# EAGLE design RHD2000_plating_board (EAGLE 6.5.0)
RHD2000 Evaluation Board

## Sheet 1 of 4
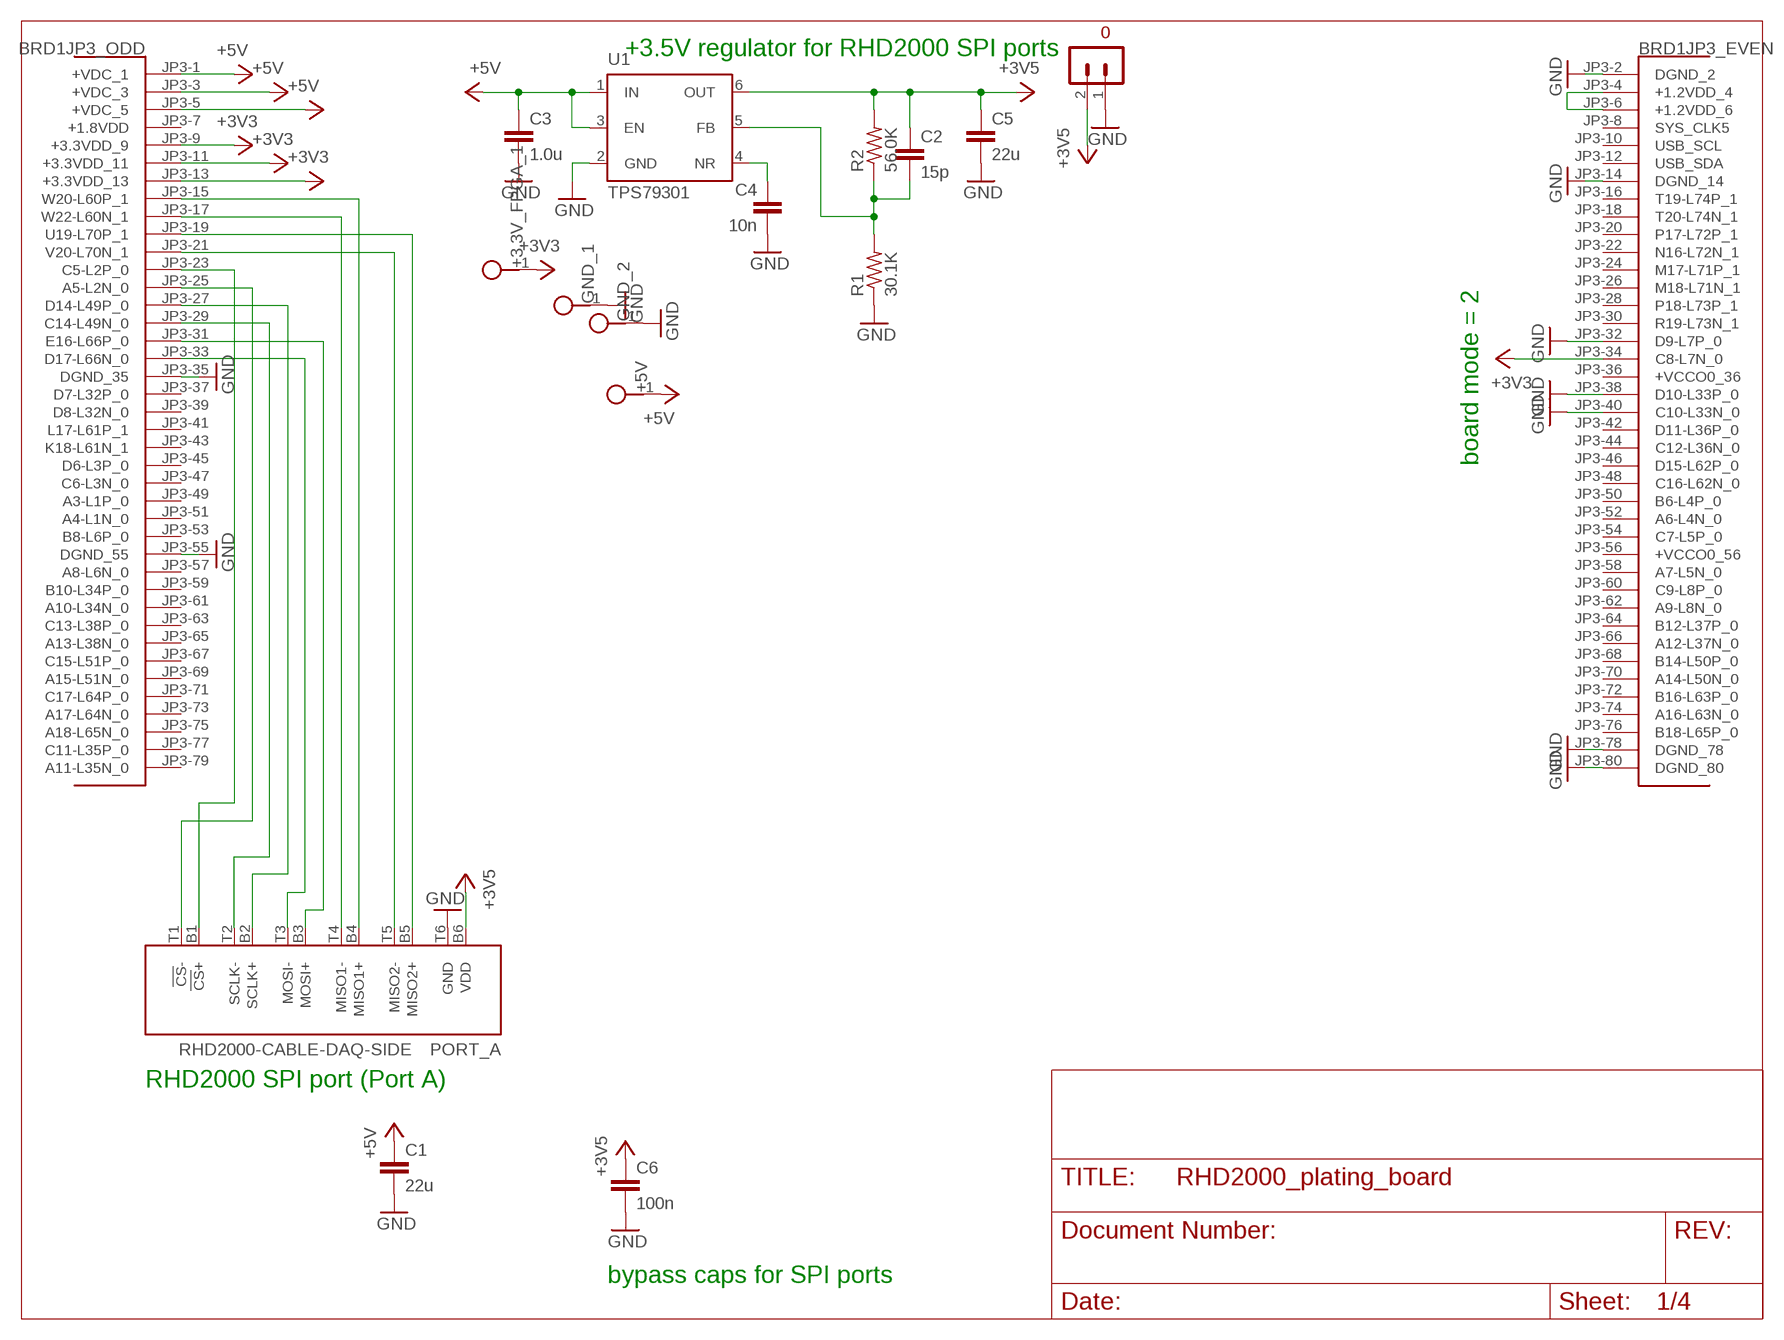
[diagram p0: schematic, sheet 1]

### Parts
+3.3V_FPGA_1  TESTPOINT  [TESTPOINT]
+5V  TESTPOINT  [TESTPOINT]
BRD1  OPALKELLY_XEM6010  [OPALKELLY_XEM6010]
C1  22u  C_1206  [1206]
C2  15p  C_0603  [0603]
C3  1.0u  C_0805  [0805]
C4  10n  C_0603  [0603]
C5  22u  C_1206  [1206]
C6  100n  C_0603  [0603]
GND_1  TESTPOINT  [TESTPOINT]
GND_2  TESTPOINT  [TESTPOINT]
PORT_A  RHD2000-CABLE-DAQ-SIDE  [OMNETICS_PZN-12-AA]
R1  30.1K  R_0603  [0603]
R2  56.0K  R_0603  [0603]
S2  TERMINAL_BLOCK_2-3.5MM-3.5V  [TERMINAL_BLOCK_3.5MM_2_3.5V]
U1  TPS79301  [SOT-23-6]

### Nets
+3V3 [power]: +3.3V_FPGA_1.1 BRD1.JP3-9(JP3_ODD:+3.3VDD_9) BRD1.JP3-11(JP3_ODD:+3.3VDD_11) BRD1.JP3-13(JP3_ODD:+3.3VDD_13) BRD1.JP3-34(JP3_EVEN:C8-L7N_0) ; also sheet 3
+3V5 [power]: C2.1 C5.1 C6.1 PORT_A.B6(VDD) R2.2 S2.2 U1.6(OUT)
+5V [power]: +5V.1 BRD1.JP3-1(JP3_ODD:+VDC_1) BRD1.JP3-3(JP3_ODD:+VDC_3) BRD1.JP3-5(JP3_ODD:+VDC_5) C1.1 C3.1 U1.1(IN) U1.3(EN) ; also sheet 4
GND [power]: BRD1.JP3-2(JP3_EVEN:DGND_2) BRD1.JP3-14(JP3_EVEN:DGND_14) BRD1.JP3-32(JP3_EVEN:D9-L7P_0) BRD1.JP3-35(JP3_ODD:DGND_35) BRD1.JP3-38(JP3_EVEN:D10-L33P_0) BRD1.JP3-40(JP3_EVEN:C10-L33N_0) BRD1.JP3-55(JP3_ODD:DGND_55) BRD1.JP3-78(JP3_EVEN:DGND_78) BRD1.JP3-80(JP3_EVEN:DGND_80) C1.2 C3.2 C4.2 C5.2 C6.2 GND_1.1 GND_2.1 PORT_A.T6(GND) R1.1 S2.1 U1.2(GND) ; also sheet 2,3,4
N$1: BRD1.JP3-15(JP3_ODD:W20-L60P_1) PORT_A.B4(MISO1+)
N$2: BRD1.JP3-17(JP3_ODD:W22-L60N_1) PORT_A.T4(MISO1-)
N$3: BRD1.JP3-19(JP3_ODD:U19-L70P_1) PORT_A.B5(MISO2+)
N$4: BRD1.JP3-21(JP3_ODD:V20-L70N_1) PORT_A.T5(MISO2-)
N$5: BRD1.JP3-23(JP3_ODD:C5-L2P_0) PORT_A.B1(!CS!+)
N$6: BRD1.JP3-25(JP3_ODD:A5-L2N_0) PORT_A.T1(!CS!-)
N$7: BRD1.JP3-27(JP3_ODD:D14-L49P_0) PORT_A.B2(SCLK+)
N$8: BRD1.JP3-29(JP3_ODD:C14-L49N_0) PORT_A.T2(SCLK-)
N$9: BRD1.JP3-31(JP3_ODD:E16-L66P_0) PORT_A.B3(MOSI+)
N$10: BRD1.JP3-33(JP3_ODD:D17-L66N_0) PORT_A.T3(MOSI-)
N$143: C4.1 U1.4(NR)
N$144: C2.2 R1.2 R2.1 U1.5(FB)
N$185 [power]: BRD1.JP3-4(JP3_EVEN:+1.2VDD_4) BRD1.JP3-6(JP3_EVEN:+1.2VDD_6)
Unconnected: BRD1.JP3-8(JP3_EVEN:SYS_CLK5) BRD1.JP3-10(JP3_EVEN:USB_SCL) BRD1.JP3-12(JP3_EVEN:USB_SDA) BRD1.JP3-16(JP3_EVEN:T19-L74P_1) BRD1.JP3-18(JP3_EVEN:T20-L74N_1) BRD1.JP3-20(JP3_EVEN:P17-L72P_1) BRD1.JP3-22(JP3_EVEN:N16-L72N_1) BRD1.JP3-24(JP3_EVEN:M17-L71P_1) BRD1.JP3-26(JP3_EVEN:M18-L71N_1) BRD1.JP3-28(JP3_EVEN:P18-L73P_1) BRD1.JP3-30(JP3_EVEN:R19-L73N_1) BRD1.JP3-37(JP3_ODD:D7-L32P_0) BRD1.JP3-39(JP3_ODD:D8-L32N_0) BRD1.JP3-41(JP3_ODD:L17-L61P_1) BRD1.JP3-42(JP3_EVEN:D11-L36P_0) BRD1.JP3-43(JP3_ODD:K18-L61N_1) BRD1.JP3-44(JP3_EVEN:C12-L36N_0) BRD1.JP3-45(JP3_ODD:D6-L3P_0) BRD1.JP3-46(JP3_EVEN:D15-L62P_0) BRD1.JP3-47(JP3_ODD:C6-L3N_0) BRD1.JP3-48(JP3_EVEN:C16-L62N_0) BRD1.JP3-49(JP3_ODD:A3-L1P_0) BRD1.JP3-50(JP3_EVEN:B6-L4P_0) BRD1.JP3-51(JP3_ODD:A4-L1N_0) BRD1.JP3-52(JP3_EVEN:A6-L4N_0) BRD1.JP3-53(JP3_ODD:B8-L6P_0) BRD1.JP3-54(JP3_EVEN:C7-L5P_0) BRD1.JP3-57(JP3_ODD:A8-L6N_0) BRD1.JP3-58(JP3_EVEN:A7-L5N_0) BRD1.JP3-59(JP3_ODD:B10-L34P_0) BRD1.JP3-60(JP3_EVEN:C9-L8P_0) BRD1.JP3-61(JP3_ODD:A10-L34N_0) BRD1.JP3-62(JP3_EVEN:A9-L8N_0) BRD1.JP3-63(JP3_ODD:C13-L38P_0) BRD1.JP3-64(JP3_EVEN:B12-L37P_0) BRD1.JP3-65(JP3_ODD:A13-L38N_0) BRD1.JP3-66(JP3_EVEN:A12-L37N_0) BRD1.JP3-67(JP3_ODD:C15-L51P_0) BRD1.JP3-68(JP3_EVEN:B14-L50P_0) BRD1.JP3-69(JP3_ODD:A15-L51N_0) BRD1.JP3-70(JP3_EVEN:A14-L50N_0) BRD1.JP3-71(JP3_ODD:C17-L64P_0) BRD1.JP3-72(JP3_EVEN:B16-L63P_0) BRD1.JP3-73(JP3_ODD:A17-L64N_0) BRD1.JP3-74(JP3_EVEN:A16-L63N_0) BRD1.JP3-75(JP3_ODD:A18-L65N_0) BRD1.JP3-76(JP3_EVEN:B18-L65P_0) BRD1.JP3-77(JP3_ODD:C11-L35P_0) BRD1.JP3-79(JP3_ODD:A11-L35N_0)

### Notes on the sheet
- +3.5V regulator for RHD2000 SPI ports
- board mode = 2
- RHD2000 SPI port (Port A)
- bypass caps for SPI ports

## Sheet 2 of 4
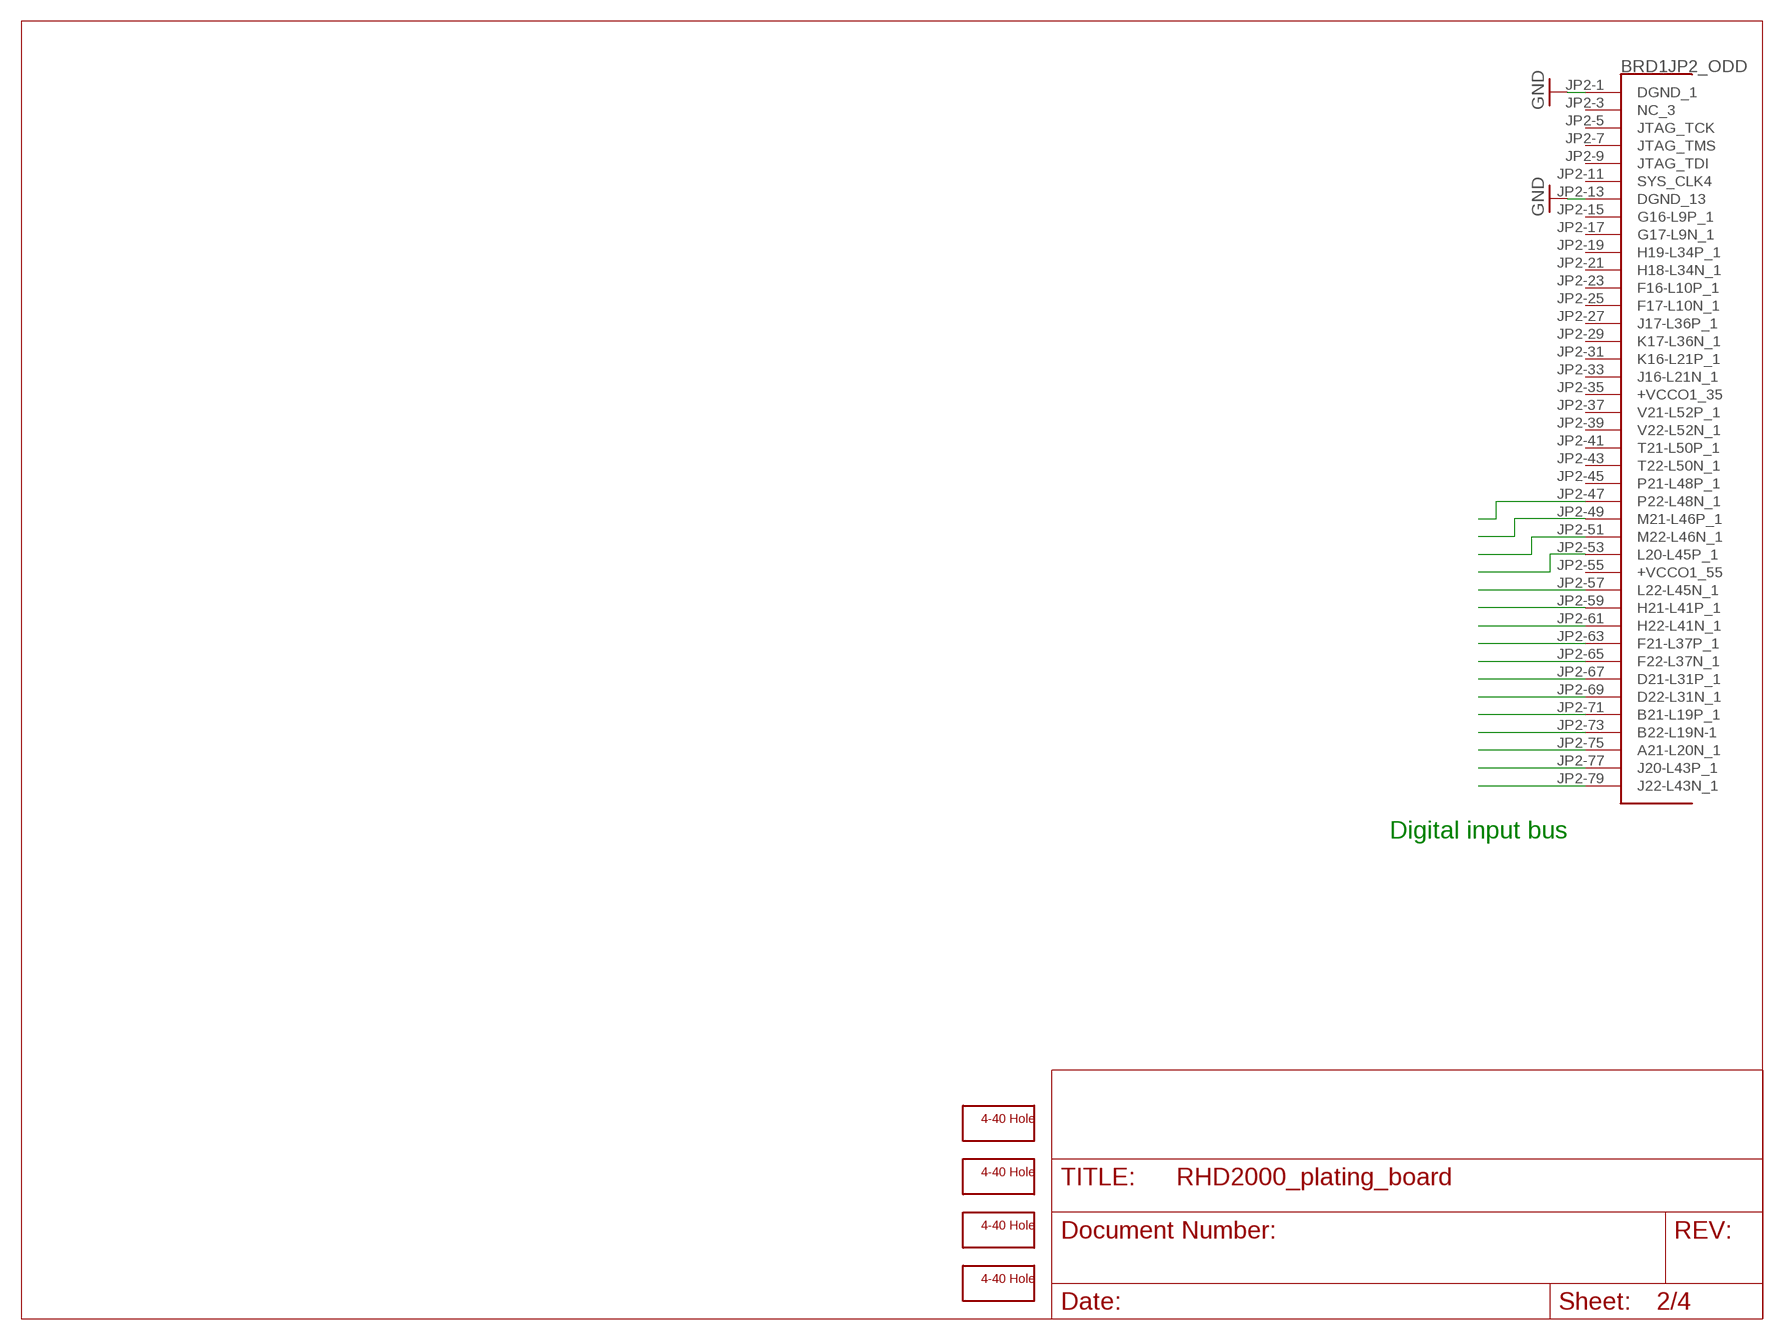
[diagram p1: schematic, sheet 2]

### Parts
H1  SCREW_HOLE_4-40  [SCREW_HOLE_4-40]
H2  SCREW_HOLE_4-40  [SCREW_HOLE_4-40]
H3  SCREW_HOLE_4-40  [SCREW_HOLE_4-40]
H4  SCREW_HOLE_4-40  [SCREW_HOLE_4-40]

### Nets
GND [power]: BRD1.JP2-1(JP2_ODD:DGND_1) BRD1.JP2-13(JP2_ODD:DGND_13) ; also sheet 1,3,4
N$68: BRD1.JP2-79(JP2_ODD:J22-L43N_1)
N$69: BRD1.JP2-77(JP2_ODD:J20-L43P_1)
N$70: BRD1.JP2-75(JP2_ODD:A21-L20N_1)
N$71: BRD1.JP2-73(JP2_ODD:B22-L19N-1)
N$72: BRD1.JP2-71(JP2_ODD:B21-L19P_1)
N$73: BRD1.JP2-69(JP2_ODD:D22-L31N_1)
N$74: BRD1.JP2-67(JP2_ODD:D21-L31P_1)
N$75: BRD1.JP2-65(JP2_ODD:F22-L37N_1)
N$76: BRD1.JP2-63(JP2_ODD:F21-L37P_1)
N$77: BRD1.JP2-61(JP2_ODD:H22-L41N_1)
N$78: BRD1.JP2-59(JP2_ODD:H21-L41P_1)
N$79: BRD1.JP2-57(JP2_ODD:L22-L45N_1)
N$80: BRD1.JP2-53(JP2_ODD:L20-L45P_1)
N$81: BRD1.JP2-51(JP2_ODD:M22-L46N_1)
N$82: BRD1.JP2-49(JP2_ODD:M21-L46P_1)
N$83: BRD1.JP2-47(JP2_ODD:P22-L48N_1)
Unconnected: BRD1.JP2-3(JP2_ODD:NC_3) BRD1.JP2-5(JP2_ODD:JTAG_TCK) BRD1.JP2-7(JP2_ODD:JTAG_TMS) BRD1.JP2-9(JP2_ODD:JTAG_TDI) BRD1.JP2-11(JP2_ODD:SYS_CLK4) BRD1.JP2-15(JP2_ODD:G16-L9P_1) BRD1.JP2-17(JP2_ODD:G17-L9N_1) BRD1.JP2-19(JP2_ODD:H19-L34P_1) BRD1.JP2-21(JP2_ODD:H18-L34N_1) BRD1.JP2-23(JP2_ODD:F16-L10P_1) BRD1.JP2-25(JP2_ODD:F17-L10N_1) BRD1.JP2-27(JP2_ODD:J17-L36P_1) BRD1.JP2-29(JP2_ODD:K17-L36N_1) BRD1.JP2-31(JP2_ODD:K16-L21P_1) BRD1.JP2-33(JP2_ODD:J16-L21N_1) BRD1.JP2-37(JP2_ODD:V21-L52P_1) BRD1.JP2-39(JP2_ODD:V22-L52N_1) BRD1.JP2-41(JP2_ODD:T21-L50P_1) BRD1.JP2-43(JP2_ODD:T22-L50N_1) BRD1.JP2-45(JP2_ODD:P21-L48P_1)

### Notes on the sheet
- Digital input bus

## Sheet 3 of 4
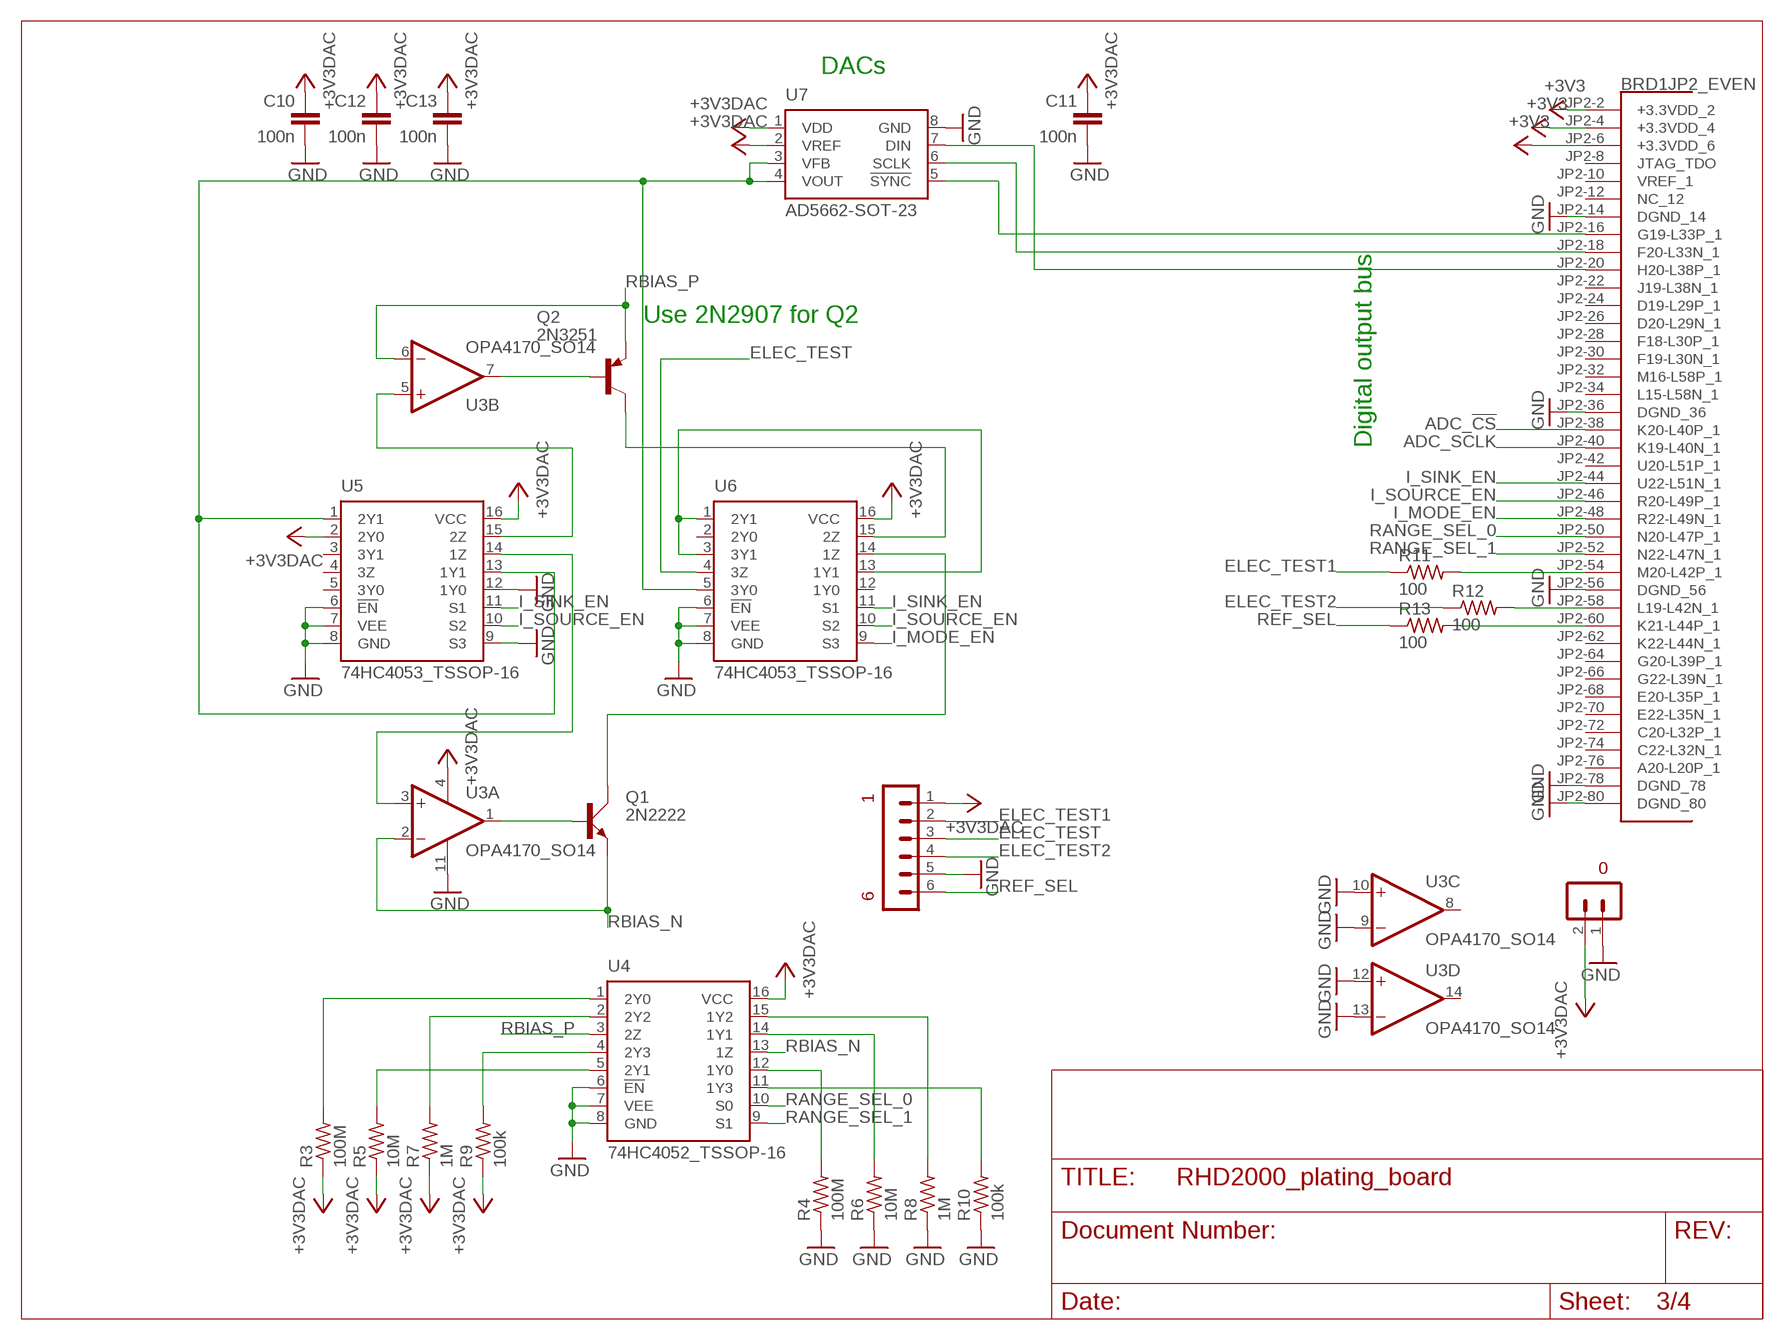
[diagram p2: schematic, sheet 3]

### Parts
C10  100n  C_0603  [0603]
C11  100n  C_0603  [0603]
C12  100n  C_0603  [0603]
C13  100n  C_0603  [0603]
Q1  2N2222  [TO18A]
Q2  2N3251  [TO18]
R3  100M  R_1206  [1206]
R4  100M  R_1206  [1206]
R5  10M  R_0603  [0603]
R6  10M  R_0603  [0603]
R7  1M  R_0603  [0603]
R8  1M  R_0603  [0603]
R9  100k  R_0603  [0603]
R10  100k  R_0603  [0603]
R11  100  R_0603  [0603]
R12  100  R_0603  [0603]
R13  100  R_0603  [0603]
S1  TERMINAL_BLOCK_2-3.5MM-3.3V  [TERMINAL_BLOCK_3.5MM_2_3.3V]
S3  WIRES-6  [WIRES-6]
U3  OPA4170_SO14  [SOIC-14]
U4  74HC4052_TSSOP-16  [TSSOP-16]
U5  74HC4053_TSSOP-16  [TSSOP-16]
U6  74HC4053_TSSOP-16  [TSSOP-16]
U7  AD5662-SOT-23  [SOT-23-RJ-8]

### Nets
+3V3 [power]: BRD1.JP2-2(JP2_EVEN:+3.3VDD_2) BRD1.JP2-4(JP2_EVEN:+3.3VDD_4) BRD1.JP2-6(JP2_EVEN:+3.3VDD_6) ; also sheet 1
+3V3DAC [power]: C10.1 C11.1 C12.1 C13.1 R3.1 R5.1 R7.1 R9.1 S1.2 S3.1 U3.4(P:V+) U4.16(VCC) U5.2(2Y0) U5.16(VCC) U6.16(VCC) U7.1(VDD) U7.2(VREF) ; also sheet 4
ADC_!CS!: BRD1.JP2-38(JP2_EVEN:K20-L40P_1)
ADC_SCLK: BRD1.JP2-40(JP2_EVEN:K19-L40N_1)
ELEC_TEST: S3.3 U6.4(3Z)
ELEC_TEST1: R11.1 S3.2
ELEC_TEST2: R12.1 S3.4
GND [power]: BRD1.JP2-14(JP2_EVEN:DGND_14) BRD1.JP2-36(JP2_EVEN:DGND_36) BRD1.JP2-56(JP2_EVEN:DGND_56) BRD1.JP2-78(JP2_EVEN:DGND_78) BRD1.JP2-80(JP2_EVEN:DGND_80) C10.2 C11.2 C12.2 C13.2 R4.1 R6.1 R8.1 R10.1 S1.1 S3.5 U3.9(C:-IN) U3.10(C:+IN) U3.11(P:V-) U3.12(D:+IN) U3.13(D:-IN) U4.6(!EN!) U4.7(VEE) U4.8(GND) U5.6(!EN!) U5.7(VEE) U5.8(GND) U5.9(S3) U5.12(1Y0) U6.6(!EN!) U6.7(VEE) U6.8(GND) U7.8(GND) ; also sheet 1,2,4
I_MODE_EN: BRD1.JP2-48(JP2_EVEN:R22-L49N_1) U6.9(S3)
I_SINK_EN: BRD1.JP2-44(JP2_EVEN:U22-L51N_1) U5.11(S1) U6.11(S1)
I_SOURCE_EN: BRD1.JP2-46(JP2_EVEN:R20-L49P_1) U5.10(S2) U6.10(S2)
N$11: Q1.B U3.1(A:OUT)
N$12: U5.1(2Y1) U5.13(1Y1) U6.5(3Y0) U7.3(VFB) U7.4(VOUT)
N$13: U3.3(A:+IN) U5.14(1Z)
N$14: Q1.C U6.14(1Z)
N$15: U3.5(B:+IN) U5.15(2Z)
N$16: Q2.2(B) U3.7(B:OUT)
N$17: Q2.3(C) U6.15(2Z)
N$18: BRD1.JP2-54(JP2_EVEN:M20-L42P_1) R11.2
N$19: BRD1.JP2-58(JP2_EVEN:L19-L42N_1) R12.2
N$20: R9.2 U4.4(2Y3)
N$21: R7.2 U4.2(2Y2)
N$22: R5.2 U4.5(2Y1)
N$23: R3.2 U4.1(2Y0)
N$24: R4.2 U4.12(1Y0)
N$25: R6.2 U4.14(1Y1)
N$26: R8.2 U4.15(1Y2)
N$27: R10.2 U4.11(1Y3)
N$28: U6.1(2Y1) U6.3(3Y1) U6.13(1Y1)
N$29: BRD1.JP2-60(JP2_EVEN:K21-L44P_1) R13.2
N$41: BRD1.JP2-16(JP2_EVEN:G19-L33P_1) U7.5(!SYNC!)
N$42: BRD1.JP2-18(JP2_EVEN:F20-L33N_1) U7.6(SCLK)
N$43: BRD1.JP2-20(JP2_EVEN:H20-L38P_1) U7.7(DIN)
RANGE_SEL_0: BRD1.JP2-50(JP2_EVEN:N20-L47P_1) U4.10(S0)
RANGE_SEL_1: BRD1.JP2-52(JP2_EVEN:N22-L47N_1) U4.9(S1)
RBIAS_N: Q1.E U3.2(A:-IN) U4.13(1Z)
RBIAS_P: Q2.1(E) U3.6(B:-IN) U4.3(2Z)
REF_SEL: R13.1 S3.6
Unconnected: BRD1.JP2-8(JP2_EVEN:JTAG_TDO) BRD1.JP2-10(JP2_EVEN:VREF_1) BRD1.JP2-12(JP2_EVEN:NC_12) BRD1.JP2-22(JP2_EVEN:J19-L38N_1) BRD1.JP2-24(JP2_EVEN:D19-L29P_1) BRD1.JP2-26(JP2_EVEN:D20-L29N_1) BRD1.JP2-28(JP2_EVEN:F18-L30P_1) BRD1.JP2-30(JP2_EVEN:F19-L30N_1) BRD1.JP2-32(JP2_EVEN:M16-L58P_1) BRD1.JP2-34(JP2_EVEN:L15-L58N_1) BRD1.JP2-42(JP2_EVEN:U20-L51P_1) BRD1.JP2-62(JP2_EVEN:K22-L44N_1) BRD1.JP2-64(JP2_EVEN:G20-L39P_1) BRD1.JP2-66(JP2_EVEN:G22-L39N_1) BRD1.JP2-68(JP2_EVEN:E20-L35P_1) BRD1.JP2-70(JP2_EVEN:E22-L35N_1) BRD1.JP2-72(JP2_EVEN:C20-L32P_1) BRD1.JP2-74(JP2_EVEN:C22-L32N_1) BRD1.JP2-76(JP2_EVEN:A20-L20P_1) U3.8(C:OUT) U3.14(D:OUT) U5.3(3Y1) U5.4(3Z) U5.5(3Y0) U6.2(2Y0) U6.12(1Y0)

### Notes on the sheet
- DACs
- Use 2N2907 for Q2
- Digital output bus

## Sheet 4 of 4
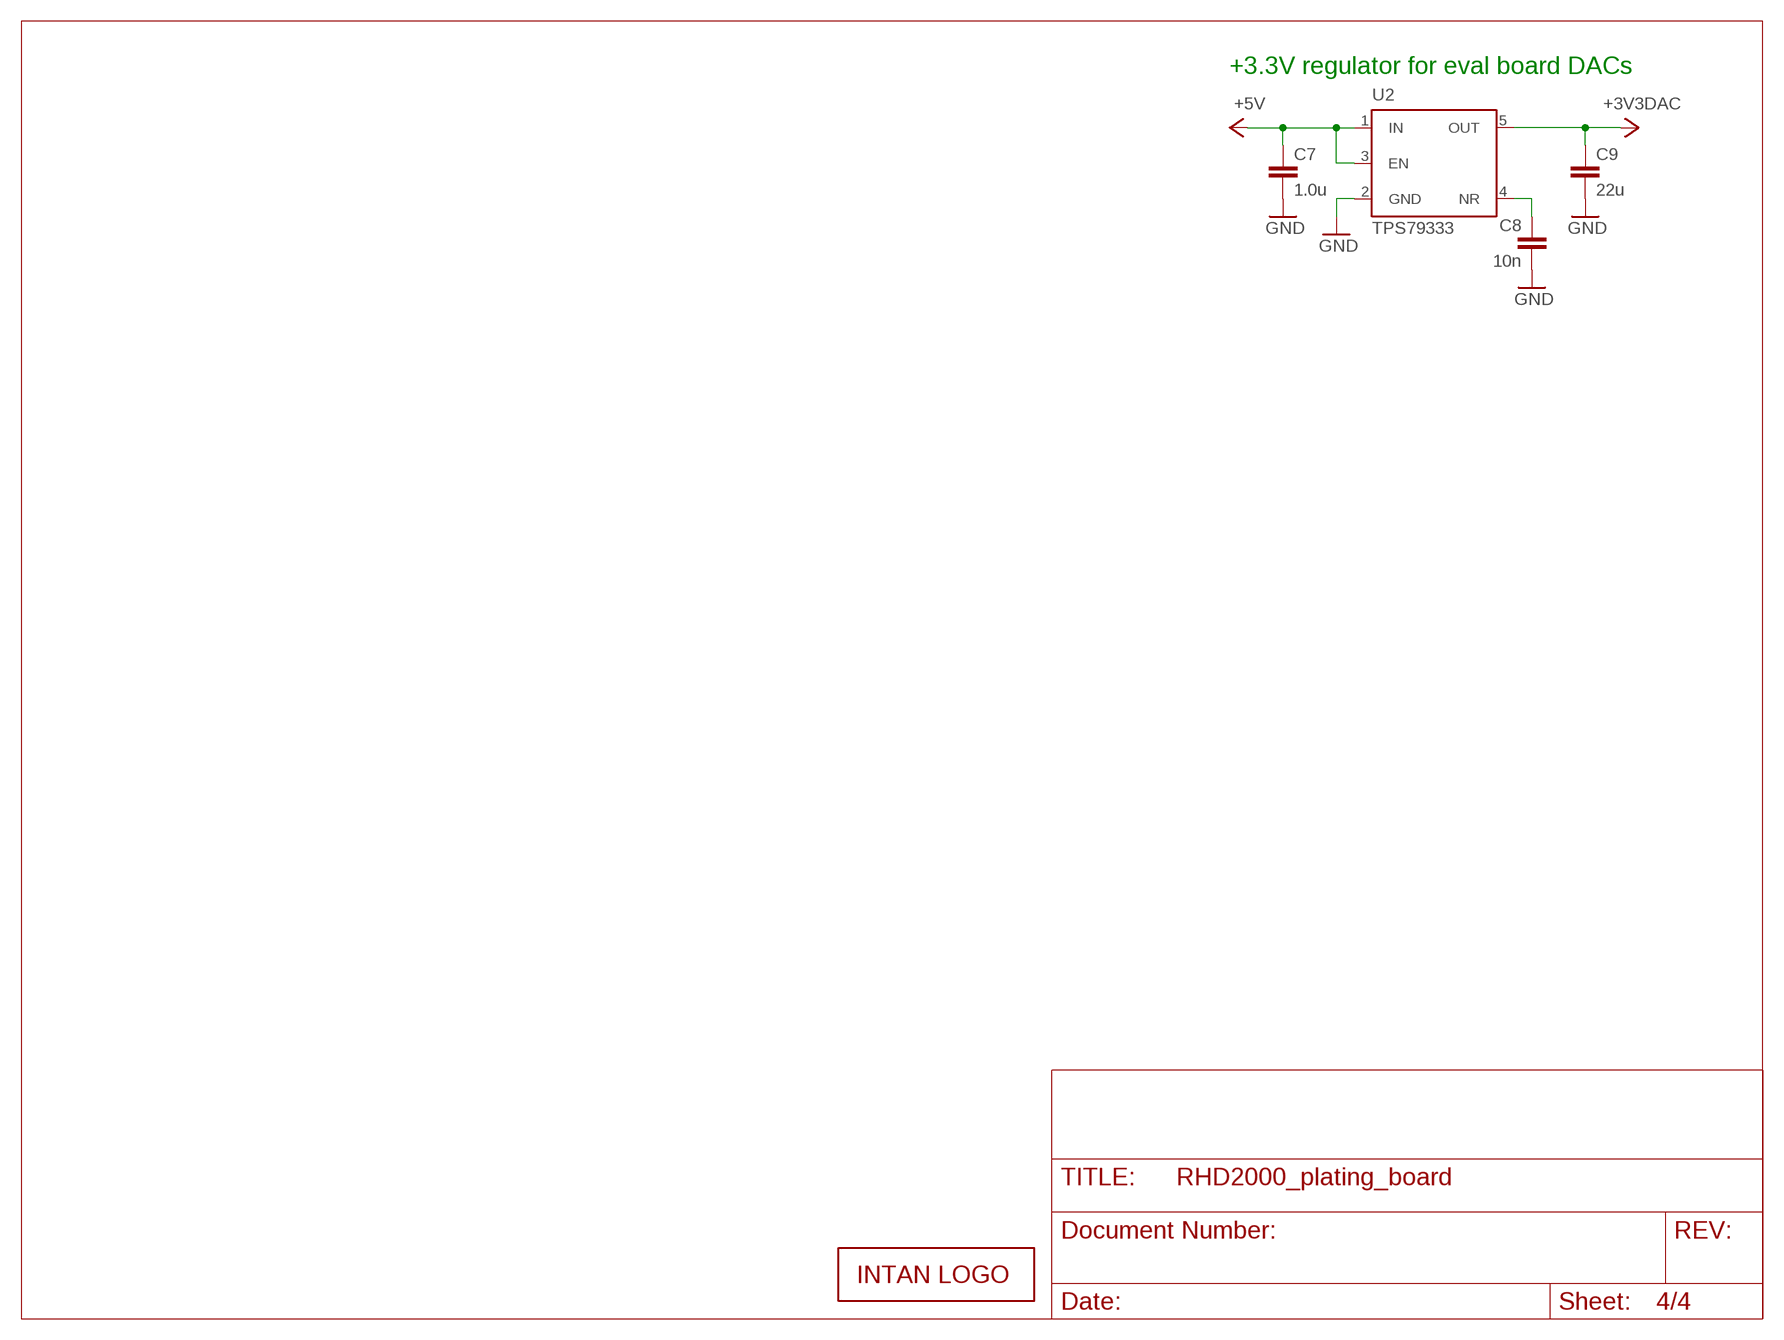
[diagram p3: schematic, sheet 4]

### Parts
C7  1.0u  C_0805  [0805]
C8  10n  C_0603  [0603]
C9  22u  C_1206  [1206]
LOGO1  INTAN_LOGO  [INTAN_LOGO]
U2  TPS79333  [SOT-23-5]

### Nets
+3V3DAC [power]: C9.1 U2.5(OUT) ; also sheet 3
+5V [power]: C7.1 U2.1(IN) U2.3(EN) ; also sheet 1
GND [power]: C7.2 C8.2 C9.2 U2.2(GND) ; also sheet 1,2,3
N$141: C8.1 U2.4(NR)

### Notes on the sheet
- +3.3V regulator for eval board DACs

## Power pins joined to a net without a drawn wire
+1.8VDD: BRD1.JP3-7(JP3_ODD:+1.8VDD)
+VCCO0_36: BRD1.JP3-36(JP3_EVEN:+VCCO0_36)
+VCCO0_56: BRD1.JP3-56(JP3_EVEN:+VCCO0_56)
+VCCO1_35: BRD1.JP2-35(JP2_ODD:+VCCO1_35)
+VCCO1_55: BRD1.JP2-55(JP2_ODD:+VCCO1_55)

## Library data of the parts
+3.3V_FPGA_1 +5V GND_1 GND_2 = RHD2000_eval_board:TESTPOINT: PCB Test Point
BRD1 = RHD2000_eval_board:OPALKELLY_XEM6010: Opal Kelly XEM6010 USB/FPGA module
C1-C13 = RHD2000_eval_board:C: Capacitor
H1-H4 = RHD2000_eval_board:SCREW_HOLE_4-40: Mounting hole
LOGO1 = RHD2000_eval_board:INTAN_LOGO
PORT_A = RHD2000_eval_board:RHD2000-CABLE-DAQ-SIDE: Omnetics PZN-12-AA RHD2000 socket - DAQ side
Q1 = transistor-small-signal:2N2222: NPN TRANSISTOR
Q2 = transistor-pnp:2N3251: PNP Transistror
R1-R13 = RHD2000_eval_board:R: Resistor
S1 S2 = RHD2000_eval_board:TERMINAL_BLOCK_2: 2-point terminal block
S3 = harrison:WIRES-6
U1 = RHD2000_eval_board:TPS79301: Texas Instruments TPS79301 adjustable regulator
U2 = RHD2000_eval_board:TPS79333: Texas Instruments TPS79333 3.3V LDO regulator
U3 = RHD2000_eval_board:OPA4170: TI OPA4170 quad op amp
U4 = harrison:74HC4052
U5 U6 = harrison:74HC4053
U7 = RHD2000_eval_board:AD5662: Analog Devices AD5662 16-bit DAC

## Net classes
1 power: width 0.381 mm

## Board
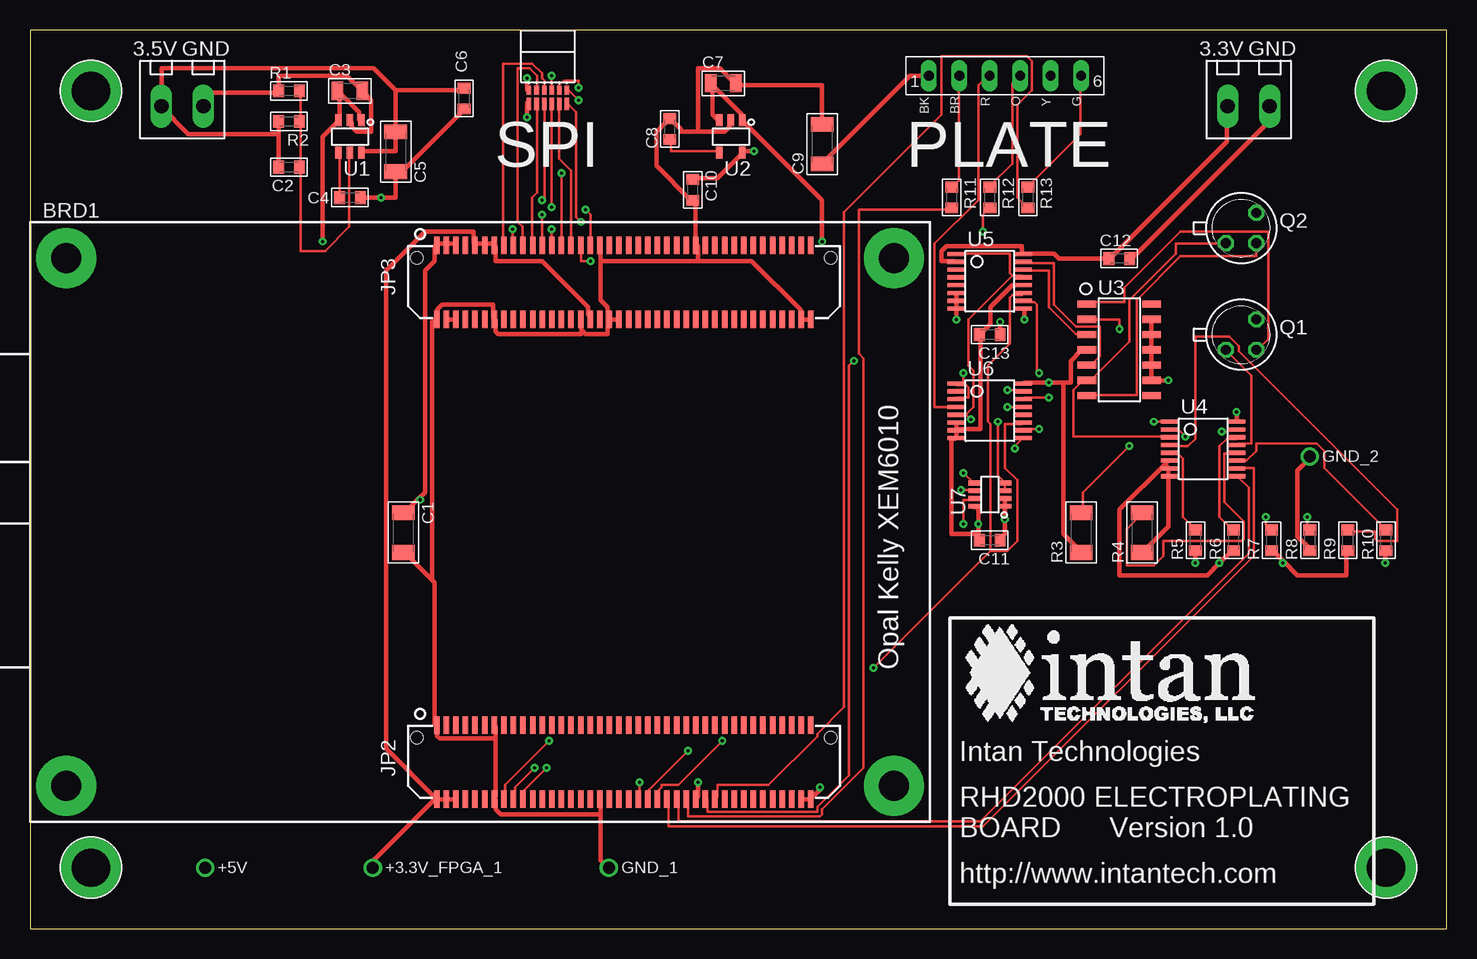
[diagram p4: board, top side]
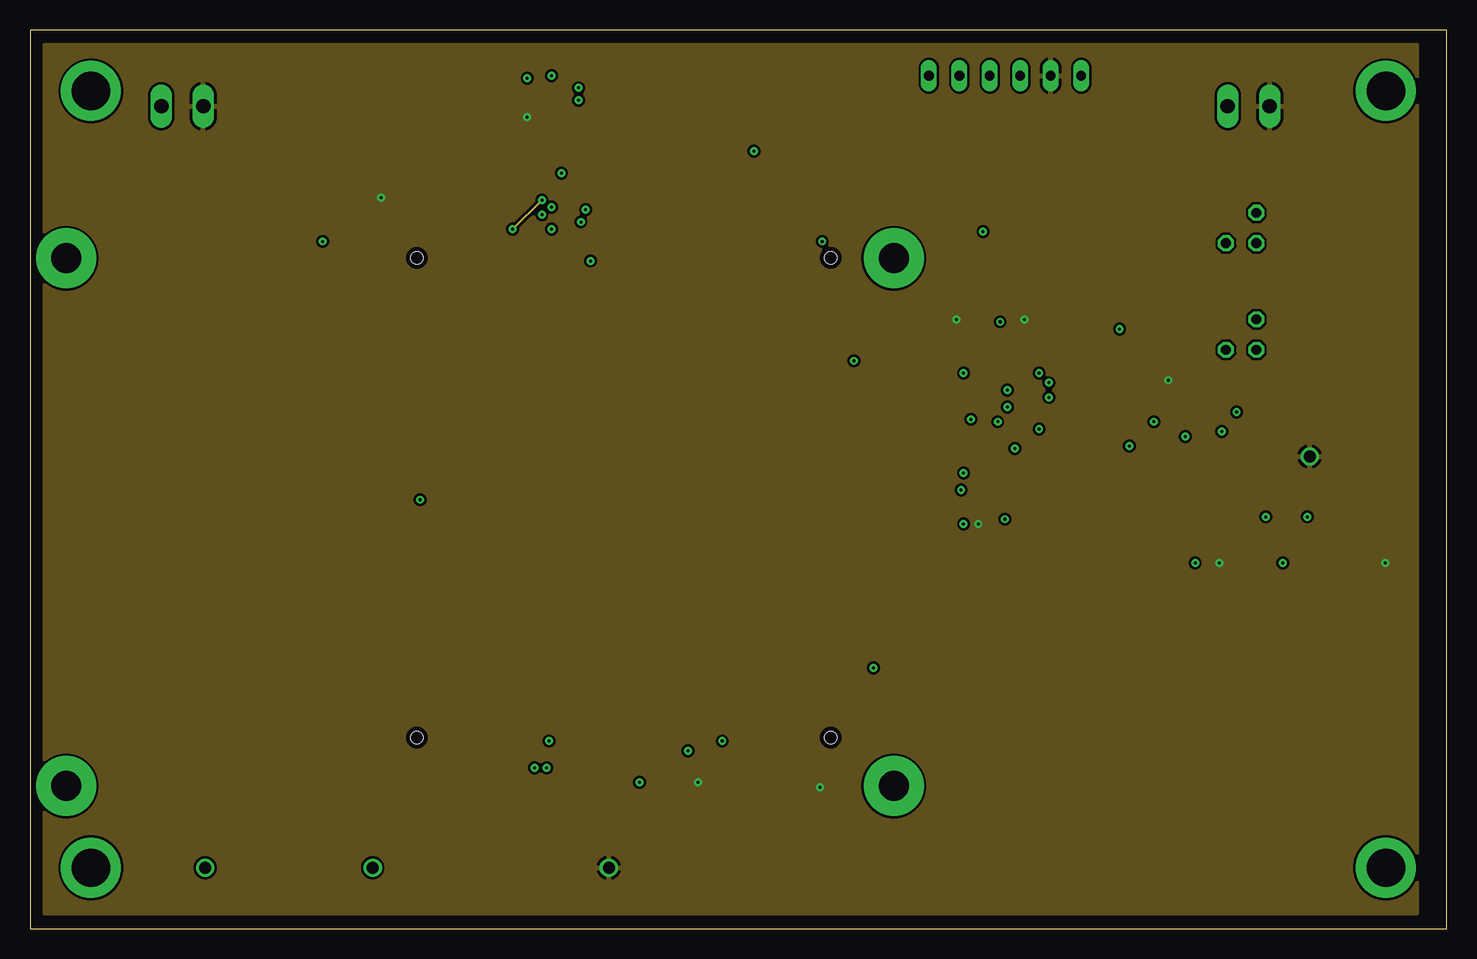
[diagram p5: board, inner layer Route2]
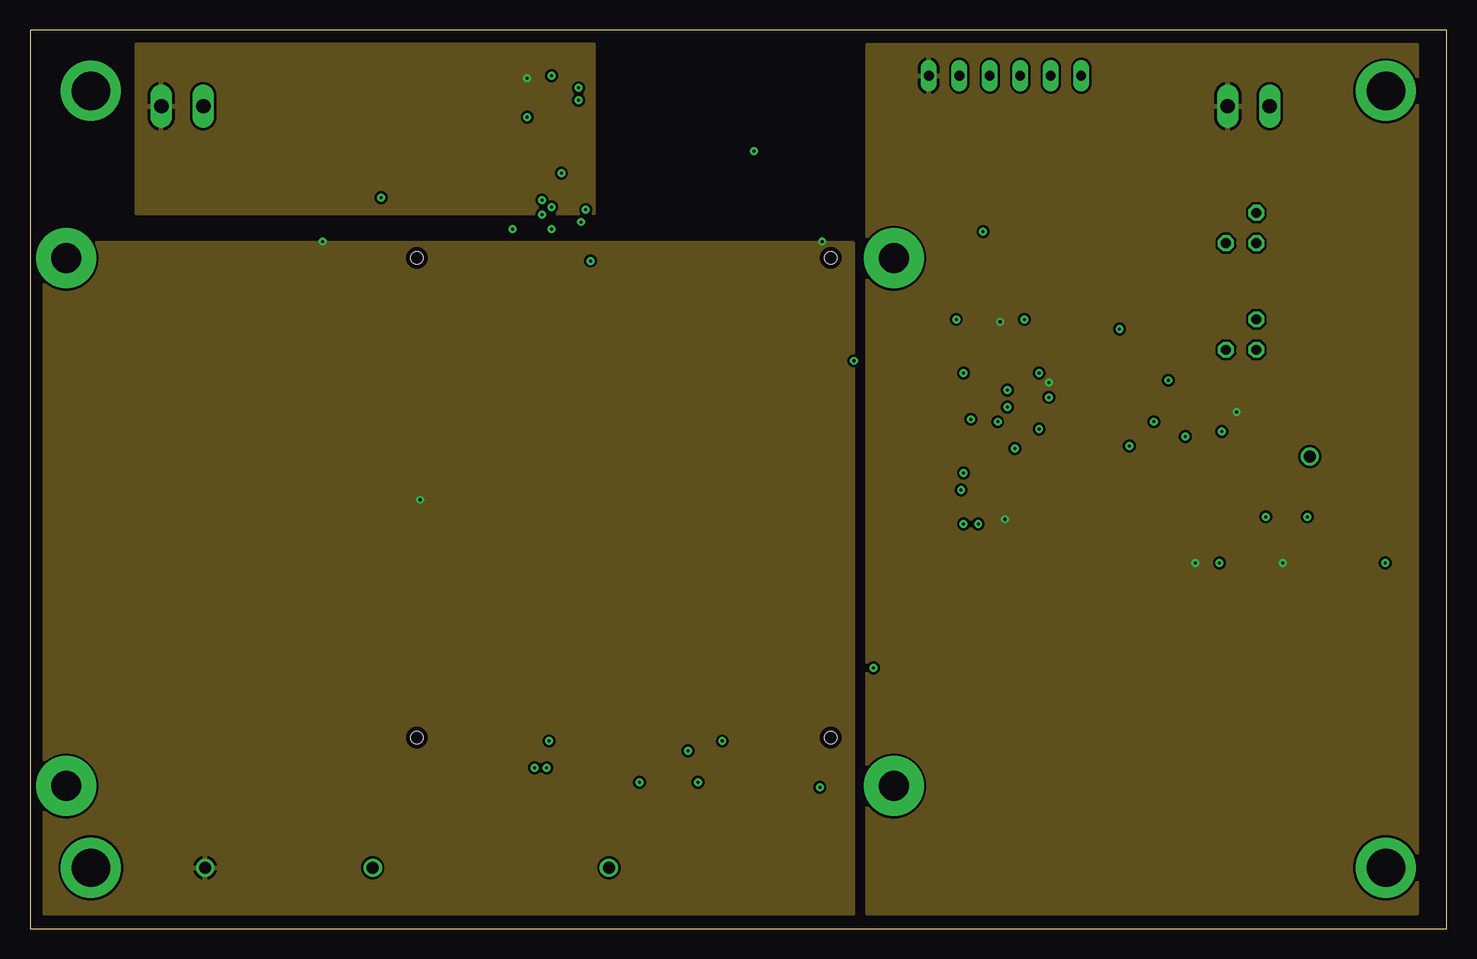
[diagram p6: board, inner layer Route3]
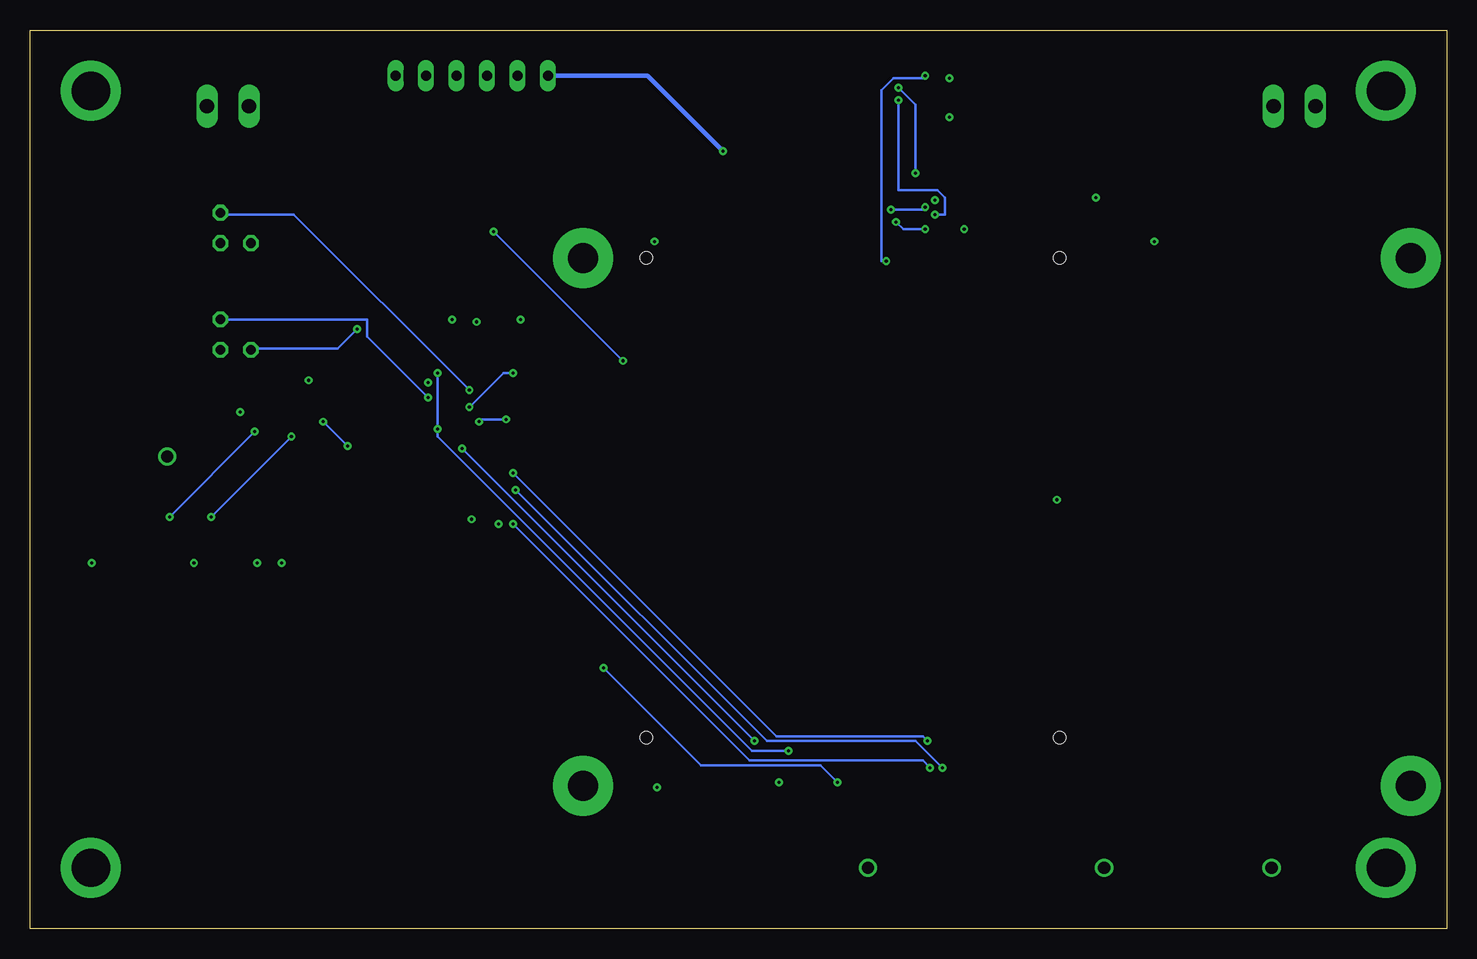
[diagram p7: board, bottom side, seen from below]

Size 118.11 x 74.93 mm. Coordinates in mm from the lower left corner, seen from the top.
Outline: 0,0 118.11,0 118.11,74.93 0,74.93 0,0
Copper layers (1*2+3*16): Top 0.035mm / dielectric 1.5mm / Route2 0.035mm / dielectric 0.15mm / Route3 0.035mm / dielectric 0.2mm / Bottom 0.035mm
Design rules "default": minimum track width 8mil, minimum drill 10mil, track to track 8mil, track to pad 8mil, pad to pad 8mil, via to via 8mil, smd to smd 8mil, copper to edge 15mil, drill to drill 8mil, minimum pad ring 10mil, minimum via ring 8mil, stop-mask expansion 4mil, vias tented up to drill 0mil, thermal gap 10mil
vRestrict: area 77.5,3.8 to 109.2,5.6; area 77.5,14 to 102.9,15.7; area 77.5,7.6 to 111.8,9.4; area 77.7,17 to 102.4,25.4; area 77.5,10.2 to 111.8,11.9; area 38.7,63.5 to 47.6,67.3; area 73,63.5 to 89.5,67.3

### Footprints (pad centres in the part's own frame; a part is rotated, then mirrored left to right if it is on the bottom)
TESTPOINT = drill 1.016: 1 0,0
OPALKELLY_XEM6010 = drill 2.5 pad 5: HOLE_NC_1 3,3; HOLE_NC_2 3,47; HOLE_NC_3 72,3; HOLE_NC_4 72,47 | smd 0.457 x 1.448: JP2-1 33.9,8.086; JP2-2 33.9,1.914; JP2-3 34.7,8.086; JP2-4 34.7,1.914; JP2-5 35.5,8.086; JP2-6 35.5,1.914; JP2-7 36.3,8.086; JP2-8 36.3,1.914; JP2-9 37.1,8.086; JP2-10 37.1,1.914; JP2-11 37.9,8.086; JP2-12 37.9,1.914; JP2-13 38.7,8.086; JP2-14 38.7,1.914; JP2-15 39.5,8.086; JP2-16 39.5,1.914; JP2-17 40.3,8.086; JP2-18 40.3,1.914; JP2-19 41.1,8.086; JP2-20 41.1,1.914; JP2-21 41.9,8.086; JP2-22 41.9,1.914; JP2-23 42.7,8.086; JP2-24 42.7,1.914; JP2-25 43.5,8.086; JP2-26 43.5,1.914; JP2-27 44.3,8.086; JP2-28 44.3,1.914; JP2-29 45.1,8.086; JP2-30 45.1,1.914; JP2-31 45.9,8.086; JP2-32 45.9,1.914; JP2-33 46.7,8.086; JP2-34 46.7,1.914; JP2-35 47.5,8.086; JP2-36 47.5,1.914; JP2-37 48.3,8.086; JP2-38 48.3,1.914; JP2-39 49.1,8.086; JP2-40 49.1,1.914; JP2-41 49.9,8.086; JP2-42 49.9,1.914; JP2-43 50.7,8.086; JP2-44 50.7,1.914; JP2-45 51.5,8.086; JP2-46 51.5,1.914; JP2-47 52.3,8.086; JP2-48 52.3,1.914; JP2-49 53.1,8.086; JP2-50 53.1,1.914; JP2-51 53.9,8.086; JP2-52 53.9,1.914; JP2-53 54.7,8.086; JP2-54 54.7,1.914; JP2-55 55.5,8.086; JP2-56 55.5,1.914; JP2-57 56.3,8.086; JP2-58 56.3,1.914; JP2-59 57.1,8.086; JP2-60 57.1,1.914; JP2-61 57.9,8.086; JP2-62 57.9,1.914; JP2-63 58.7,8.086; JP2-64 58.7,1.914; JP2-65 59.5,8.086; JP2-66 59.5,1.914; JP2-67 60.3,8.086; JP2-68 60.3,1.914; JP2-69 61.1,8.086; JP2-70 61.1,1.914; JP2-71 61.9,8.086; JP2-72 61.9,1.914; JP2-73 62.7,8.086; JP2-74 62.7,1.914; JP2-75 63.5,8.086; JP2-76 63.5,1.914; JP2-77 64.3,8.086; JP2-78 64.3,1.914; JP2-79 65.1,8.086; JP2-80 65.1,1.914; JP3-1 33.9,48.086; JP3-2 33.9,41.914; JP3-3 34.7,48.086; JP3-4 34.7,41.914; JP3-5 35.5,48.086; JP3-6 35.5,41.914; JP3-7 36.3,48.086; JP3-8 36.3,41.914; JP3-9 37.1,48.086; JP3-10 37.1,41.914; JP3-11 37.9,48.086; JP3-12 37.9,41.914; JP3-13 38.7,48.086; JP3-14 38.7,41.914; JP3-15 39.5,48.086; JP3-16 39.5,41.914; JP3-17 40.3,48.086; JP3-18 40.3,41.914; JP3-19 41.1,48.086; JP3-20 41.1,41.914; JP3-21 41.9,48.086; JP3-22 41.9,41.914; JP3-23 42.7,48.086; JP3-24 42.7,41.914; JP3-25 43.5,48.086; JP3-26 43.5,41.914; JP3-27 44.3,48.086; JP3-28 44.3,41.914; JP3-29 45.1,48.086; JP3-30 45.1,41.914; JP3-31 45.9,48.086; JP3-32 45.9,41.914; JP3-33 46.7,48.086; JP3-34 46.7,41.914; JP3-35 47.5,48.086; JP3-36 47.5,41.914; JP3-37 48.3,48.086; JP3-38 48.3,41.914; JP3-39 49.1,48.086; JP3-40 49.1,41.914; JP3-41 49.9,48.086; JP3-42 49.9,41.914; JP3-43 50.7,48.086; JP3-44 50.7,41.914; JP3-45 51.5,48.086; JP3-46 51.5,41.914; JP3-47 52.3,48.086; JP3-48 52.3,41.914; JP3-49 53.1,48.086; JP3-50 53.1,41.914; JP3-51 53.9,48.086; JP3-52 53.9,41.914; JP3-53 54.7,48.086; JP3-54 54.7,41.914; JP3-55 55.5,48.086; JP3-56 55.5,41.914; JP3-57 56.3,48.086; JP3-58 56.3,41.914; JP3-59 57.1,48.086; JP3-60 57.1,41.914; JP3-61 57.9,48.086; JP3-62 57.9,41.914; JP3-63 58.7,48.086; JP3-64 58.7,41.914; JP3-65 59.5,48.086; JP3-66 59.5,41.914; JP3-67 60.3,48.086; JP3-68 60.3,41.914; JP3-69 61.1,48.086; JP3-70 61.1,41.914; JP3-71 61.9,48.086; JP3-72 61.9,41.914; JP3-73 62.7,48.086; JP3-74 62.7,41.914; JP3-75 63.5,48.086; JP3-76 63.5,41.914; JP3-77 64.3,48.086; JP3-78 64.3,41.914; JP3-79 65.1,48.086; JP3-80 65.1,41.914 | hole 1.016: 32.261,47.032; 66.739,47.032; 32.261,7.032; 66.739,7.032
1206 = smd 1.219 x 1.88: 1 -1.651,0; 2 1.651,0
0603 = smd 0.889 x 1.067: 1 -0.864,0; 2 0.864,0
0805 = smd 0.965 x 1.524: 1 -1.041,0; 2 1.041,0
SCREW_HOLE_4-40 = drill 3.2 pad 5: 1 0,0
OMNETICS_PZN-12-AA = smd 0.381 x 0.762: B1 1.587,-1.016; B2 0.953,-1.016; B3 0.318,-1.016; B4 -0.318,-1.016; B5 -0.953,-1.016; B6 -1.587,-1.016 | smd 0.381 x 1.016: T1 1.587,-2.159; T2 0.953,-2.159; T3 0.318,-2.159; T4 -0.318,-2.159; T5 -0.953,-2.159; T6 -1.587,-2.159
TO18A = drill 0.813 octagon: B 1.27,-1.27; C 1.27,1.27; E -1.27,-1.27
TO18 = drill 0.813 octagon: 1 -1.27,-1.27; 2 1.27,-1.27; 3 1.27,1.27
TERMINAL_BLOCK_3.5MM_2_3.3V = drill 1.2 long: 1 -1.75,0; 2 1.75,0
TERMINAL_BLOCK_3.5MM_2_3.5V = drill 1.2 long: 1 -1.75,0; 2 1.75,0
WIRES-6 = drill 0.813 long: 1 -6.35,0; 2 -3.81,0; 3 -1.27,0; 4 1.27,0; 5 3.81,0; 6 6.35,0
SOT-23-6 = smd 0.55 x 1: 1 -0.95,-1.35; 2 0,-1.35; 3 0.95,-1.35; 4 0.95,1.35; 5 0,1.35; 6 -0.95,1.35
SOT-23-5 = smd 0.55 x 1: 1 -0.95,-1.35; 2 0,-1.35; 3 0.95,-1.35; 4 0.95,1.35; 5 -0.95,1.35
SOIC-14 = smd 0.6 x 1.55: 1 -3.81,-2.7; 2 -2.54,-2.7; 3 -1.27,-2.7; 4 0,-2.7; 5 1.27,-2.7; 6 2.54,-2.7; 7 3.81,-2.7; 8 3.81,2.7; 9 2.54,2.7; 10 1.27,2.7; 11 0,2.7; 12 -1.27,2.7; 13 -2.54,2.7; 14 -3.81,2.7
TSSOP-16 = smd 0.348 x 1.397: 1 -2.273,-2.814; 2 -1.623,-2.815; 3 -0.973,-2.815; 4 -0.323,-2.815; 5 0.327,-2.815; 6 0.977,-2.815; 7 1.627,-2.815; 8 2.277,-2.815; 9 2.277,2.825; 10 1.627,2.825; 11 0.977,2.825; 12 0.327,2.825; 13 -0.323,2.825; 14 -0.973,2.825; 15 -1.623,2.825; 16 -2.273,2.825
SOT-23-RJ-8 = smd 0.4 x 1: 1 -0.975,-1.3; 2 -0.325,-1.3; 3 0.325,-1.3; 4 0.975,-1.3; 5 0.975,1.3; 6 0.325,1.3; 7 -0.325,1.3; 8 -0.975,1.3

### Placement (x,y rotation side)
+3.3V_FPGA_1  28.57,5.08 0 top
+5V  14.61,5.08 0 top
BRD1  0,8.89 0 top
C1  31.11,33.02 270 top
C2  21.59,63.5 0 top
C3  26.67,69.85 0 top
C4  26.67,60.96 0 top
C5  30.48,64.77 270 top
C6  36.2,69.22 270 top
C7  57.78,70.48 0 top
C8  53.34,66.67 90 top
C9  66.04,65.41 90 top
C10  55.24,61.59 270 top
C11  80.01,32.38 180 top
C12  90.81,55.88 0 top
C13  80.01,49.53 180 top
GND_1  48.26,5.08 0 top
GND_2  106.68,39.37 0 top
H1  5.08,69.85 0 top
H2  113.03,69.85 0 top
H3  113.03,5.08 0 top
H4  5.08,5.08 0 top
LOGO1  77.47,16.51 0 top
PORT_A  43.18,70.92 0 top
Q1  100.97,49.53 0 top
Q2  100.97,58.42 0 top
R1  21.59,69.85 0 top
R2  21.59,67.31 180 top
R3  87.63,33.02 90 top
R4  92.71,33.02 90 top
R5  97.16,32.38 90 top
R6  100.33,32.38 90 top
R7  103.5,32.38 90 top
R8  106.68,32.38 90 top
R9  109.86,32.38 90 top
R10  113.03,32.38 90 top
R11  76.83,60.96 270 top
R12  80.01,60.96 270 top
R13  83.19,60.96 270 top
S1  101.6,68.58 180 top
S2  12.7,68.58 180 top
S3  81.28,71.12 0 top
U1  26.67,66.04 180 top
U2  58.42,66.04 180 top
U3  90.81,48.26 270 top
U4  97.79,40.01 270 top
U5  80.01,53.98 270 top
U6  80.01,43.18 270 top
U7  80.01,36.2 90 top

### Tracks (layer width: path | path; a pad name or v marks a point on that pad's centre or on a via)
+3V3
  Top 0.381: BRD1.JP2-2 33.93,10.77 34.54,10.77 BRD1.JP2-4 34.75,10.77 35.36,10.77 BRD1.JP2-6 | BRD1.JP2-2 33.73,10.77 28.65,5.69 28.65,5.08 +3.3V_FPGA_1.1 | BRD1.JP3-34 46.74,51 46.53,51.21 46.53,51.82 42.67,55.68 38.81,55.68 38.81,56.9 BRD1.JP3-13 38.61,57.1 38,57.1 BRD1.JP3-11 37.8,57.1 37.19,57.1 BRD1.JP3-9 36.98,57.1 36.98,58.12 32.92,58.12 29.67,54.86 29.67,15.04 BRD1.JP2-2
+3V3DAC  (via drill 0.25)
  Top 0.381: 86.16,45.52 86.77,45.52 86.77,47.35 87.58,48.16 87.99,48.16 U3.4 | 86.16,45.52 v84.94,45.52 82.91,45.52 U6.16 | 86.16,45.52 86.16,32.92 87.58,31.5 R3.1 | U5.2 77.01,55.68 76,55.68 76,56.49 76.4,56.9 82.7,56.9 82.7,56.29 U5.16 82.91,56.29 85.34,56.29 85.75,55.88 C12.1 90.02,55.88 99.77,65.63 99.77,68.48 S1.2 | 104.55,30.58 105.66,29.46 109.73,29.46 109.73,31.5 R9.1 | 104.55,30.58 103.63,31.5 R7.1 | C10.1 55.27,62.59 57.3,62.59 59.33,64.62 U2.5 59.54,64.82 v60.35,64.82 | U7.2 81.28,35.76 81.28,35.36 U7.1 81.28,35.15 v81.28,34.14 81.28,32.92 80.87,32.51 C11.1 | v80.87,50.6 C13.1 | v97.13,30.48 97.13,31.5 R5.1 | v100.58,43.08 100.58,42.27 U4.16 | S3.1 73.36,71.12 66.04,63.8 C9.1 | v104.44,30.48 104.55,30.58
  Bottom 0.381: v60.35,64.82 66.65,71.12 S3.1
  pour Route3: 69.85,1.27 69.85,73.66 115.57,73.66 115.57,1.27
+3V5  (via drill 0.25)
  Top 0.381: U1.6 27.64,64.82 30.48,64.82 C5.1 30.48,69.9 | 30.48,69.9 36.17,69.9 C6.1 | v41.45,70.92 41.45,69.9 PORT_A.B6 | 20.73,66.24 13.21,66.24 10.97,68.48 S2.2 10.97,68.68 10.97,71.73 28.65,71.73 30.48,69.9 | R2.2 20.73,66.24 | 20.73,66.24 C2.1
  pour Route3: 8.89,73.66 8.89,59.69 46.99,59.69 46.99,73.66
+5V  (via drill 0.25)
  Top 0.381: BRD1.JP3-5 35.36,57.1 34.75,57.1 BRD1.JP3-3 34.54,57.1 33.93,57.1 BRD1.JP3-1 33.73,56.9 33.73,55.68 32.92,54.86 32.92,36.37 32.41,35.87 | 32.41,35.87 31.29,34.75 C1.1 | 56.9,70.31 56.9,67.87 57.3,67.46 U2.3 | 56.9,70.31 59.33,67.87 59.33,67.46 U2.1 59.54,67.26 66.04,60.76 v66.04,57.3 | 56.9,70.31 C7.1 | 25.81,69.7 25.81,67.46 U1.3 25.6,67.26 24.38,66.04 v24.38,57.3 | 25.81,69.7 27.43,68.07 27.43,67.46 U1.1 | 25.81,69.7 C3.1 | v32.51,35.76 32.41,35.87
  Route3 0.381: v24.38,57.3 24.38,57.15 | v66.04,57.3 66.04,57.15
  pour Route3: 1.27,1.27 1.27,57.15 68.58,57.15 68.58,1.27
ELEC_TEST
  Top 0.203: U6.4 77.01,43.48 75.39,43.48 75.39,57.1 79.05,60.76 79.05,70.31 79.86,71.12 S3.3
ELEC_TEST1
  Top 0.203: R11.1 77.01,61.98 77.42,62.38 77.42,71.12 S3.2
ELEC_TEST2
  Top 0.203: R12.1 80.06,61.98 81.89,63.8 81.89,70.51 82.5,71.12 S3.4
GND  (via drill 0.25)
  Top 0.381: 46.02,49.89 46.33,49.58 48.16,49.58 48.16,50.8 BRD1.JP3-38 | 46.02,49.89 45.92,49.99 45.92,50.8 BRD1.JP3-32 | BRD1.JP3-40 48.97,50.8 48.36,50.8 BRD1.JP3-38 | 47.55,55.68 47.55,52.43 48.16,51.82 48.16,51 BRD1.JP3-38 | 47.55,55.68 47.55,56.9 BRD1.JP3-35 | 46.02,49.89 45.92,49.78 45.92,49.58 39.01,49.58 38.81,49.78 38.81,50.8 BRD1.JP3-14 38.61,51 38.61,52.02 34.34,52.02 33.93,51.61 33.93,51 BRD1.JP3-2 33.73,50.8 33.53,50.6 33.53,29.26 33.43,29.16 | C9.2 66.04,70.31 58.93,70.31 C7.2 58.73,70.51 57.51,71.73 55.68,71.73 55.68,66.45 | 58.52,67.46 U2.2 58.32,67.26 58.32,66.85 57.91,66.45 55.68,66.45 | 55.68,66.45 54.25,66.45 54.25,66.65 53.44,67.46 C8.2 53.24,67.46 52.22,66.45 52.22,63.6 55.07,60.76 C10.2 55.27,60.55 55.47,60.35 55.47,57.1 BRD1.JP3-55 55.68,56.9 55.68,55.68 | BRD1.JP3-80 65.02,50.8 64.41,50.8 BRD1.JP3-78 64.21,51 64.21,51.61 60.15,55.68 55.68,55.68 | 55.68,55.68 47.55,55.68 | 38.81,15.85 38.81,16.87 BRD1.JP2-13 | 38.81,15.85 38.81,10.97 BRD1.JP2-14 38.81,10.77 38.81,9.96 39.22,9.55 47.55,9.55 | 38.81,15.85 34.14,15.85 33.93,16.05 33.93,16.87 BRD1.JP2-1 33.73,17.07 33.73,28.85 33.43,29.16 | 33.43,29.16 31.29,31.29 C1.2 | 78.64,35.15 U7.8 78.84,35.15 79.05,34.95 v79.05,33.73 79.05,32.92 | 79.05,32.92 79.05,32.51 C11.2 | 77.22,41.66 77.22,42.06 U6.6 | U5.12 82.7,53.65 81.89,53.65 80.06,51.82 80.06,50.39 79.25,49.58 C13.2 79.25,49.38 79.25,41.66 77.22,41.66 | 77.22,41.66 U6.7 77.22,41.45 77.22,41.05 U6.8 77.01,40.84 76.81,40.64 76.81,32.92 79.05,32.92 | 94.89,38.41 94.89,37.8 U4.8 94.89,37.59 94.89,33.53 92.86,31.5 R4.1 | 94.59,38.71 94.89,39.01 U4.6
  Top 0.381: 94.59,38.71 90.83,34.95 90.83,29.46 98.15,29.46 v99.16,30.48 100.18,31.5 R6.1 | 94.59,38.71 94.89,38.41 | 94.89,38.41 U4.7 | C4.2 v29.26,60.96 30.48,60.96 30.48,62.59 | 30.48,62.59 C5.2 30.48,62.99 | 30.48,62.59 36.17,68.28 C6.2 | U3.13 93.47,50.8 93.47,49.58 U3.12 93.47,49.38 93.47,48.36 U3.11 93.47,48.16 93.47,47.14 U3.10 93.47,46.94 93.47,45.72 U3.9 v94.89,45.72 | 26.62,67.46 U1.2 26.82,67.26 26.82,66.85 27.23,66.45 28.45,66.45 28.45,69.09 27.84,69.7 C3.2 27.64,69.9 26.42,71.12 20.73,71.12 R1.1 20.73,69.7 14.63,69.7 14.63,68.68 S2.1 | U5.6 77.22,52.83 77.22,52.43 U5.7 77.22,52.22 77.22,51.82 U5.8 77.22,51.61 v77.22,50.8 | BRD1.JP2-78 64.41,10.77 65.02,10.77 BRD1.JP2-80 65.23,10.97 65.84,11.58 v65.84,11.79 | 41.45,68.89 PORT_A.T6 41.45,68.68 v41.45,67.67 | R8.1 106.68,31.7 105.66,32.72 105.66,38.2 106.68,39.22 GND_2.1 | v112.98,30.48 112.98,31.5 R10.1 | C12.2 91.85,55.88 103.23,67.26 103.23,68.48 S1.1 | v82.91,50.8 82.91,51.61 U5.9 | 47.55,9.55 47.55,5.69 48.16,5.08 GND_1.1 | 47.55,9.55 47.55,10.77 BRD1.JP2-36 | v55.68,12.19 55.68,10.97 BRD1.JP2-56
  pour Route2: 1.27,73.66 115.57,73.66 115.57,1.27 1.27,1.27
I_MODE_EN  (via drill 0.25)
  Top 0.203: v82.09,40.03 82.09,40.23 82.7,40.84 U6.9 | v57.71,15.65 54.05,11.99 52.63,11.99 52.63,11.79 52.43,11.58 52.43,10.97 BRD1.JP2-48
  Bottom 0.203: v57.71,15.65 v82.09,40.03
I_SINK_EN  (via drill 0.25)
  Top 0.203: 80.06,31.5 81.48,31.5 82.3,32.31 82.3,37.39 81.28,38.41 81.28,42.06 82.7,42.06 U6.11 | 80.06,31.5 80.06,42.06 79.86,42.27 79.86,46.94 81.69,48.77 81.69,52.63 81.89,52.83 82.7,52.83 U5.11 | v50.8,12.19 50.8,10.97 BRD1.JP2-44 | 80.06,31.5 v70.31,21.74
  Bottom 0.203: v50.8,12.19 52.22,13.61 62.18,13.61 v70.31,21.74
I_SOURCE_EN  (via drill 0.25)
  Top 0.203: v84.12,41.66 82.91,41.66 U6.10 | v84.12,46.33 83.92,46.53 83.92,52.02 83.72,52.22 82.91,52.22 U5.10 | v54.86,14.83 51.61,11.58 51.61,10.97 BRD1.JP2-46
  Bottom 0.203: v84.12,46.33 v84.12,41.66 84.12,41.05 57.91,14.83 v54.86,14.83
N$1
  Top 0.203: PORT_A.B4 42.88,69.9 42.88,70.71 42.67,70.92 42.67,71.32 41.86,72.14 39.42,72.14 39.42,57.1 BRD1.JP3-15
N$2  (via drill 0.25)
  Top 0.203: v42.67,60.76 42.88,60.96 42.88,68.68 PORT_A.T4 | v40.23,58.32 40.23,57.1 BRD1.JP3-17
  Route2 0.203: v40.23,58.32 v42.67,60.76
N$3
  Top 0.203: PORT_A.B5 42.27,69.9 42.27,71.12 41.66,71.73 40.64,71.73 40.64,58.93 41.05,58.52 41.05,57.1 BRD1.JP3-19
N$4
  Top 0.203: PORT_A.T5 42.27,68.68 42.27,61.37 41.86,60.96 41.86,57.1 BRD1.JP3-21
N$5  (via drill 0.25)
  Top 0.203: v45.72,69.09 44.91,69.9 PORT_A.B1 | v42.67,59.54 42.67,57.1 BRD1.JP3-23
  Bottom 0.203: v45.72,69.09 45.72,61.57 42.47,61.57 41.86,60.96 41.86,59.54 v42.67,59.54
N$6  (via drill 0.25)
  Top 0.203: v45.92,58.93 45.52,59.33 45.52,68.07 44.91,68.68 PORT_A.T1 | v43.48,58.32 43.48,57.1 BRD1.JP3-25
  Bottom 0.203: v45.92,58.93 45.31,58.32 v43.48,58.32
N$7  (via drill 0.25)
  Top 0.203: v45.72,70.1 45.72,70.71 44.5,70.71 44.09,70.31 44.09,69.9 PORT_A.B2 | v44.3,62.99 44.3,57.1 BRD1.JP3-27
  Bottom 0.203: v45.72,70.1 44.3,68.68 v44.3,62.99
N$8
  Top 0.203: PORT_A.T2 44.09,68.68 44.09,64.21 45.11,63.2 45.11,57.1 BRD1.JP3-29
N$9  (via drill 0.25)
  Top 0.203: v43.48,71.12 43.48,69.9 PORT_A.B3 | v46.74,55.68 45.92,55.68 45.92,56.9 BRD1.JP3-31
  Bottom 0.203: v43.48,71.12 43.69,70.92 46.13,70.92 47.14,69.9 47.14,55.68 v46.74,55.68
N$10  (via drill 0.25)
  Top 0.203: v43.48,60.15 43.48,68.68 PORT_A.T3 | v46.33,59.94 46.74,59.54 46.74,57.1 BRD1.JP3-33
  Bottom 0.203: v43.48,60.15 43.69,59.94 v46.33,59.94
N$11
  Top 0.203: U3.1 88.19,52.22 91.24,52.22 91.24,53.44 95.91,58.12 103.23,58.12 103.23,49.17 102.41,48.36 Q1.B
N$12  (via drill 0.25)
  Top 0.203: 81.89,54.46 81.69,54.66 81.69,56.29 77.22,56.29 U5.1 | 81.89,54.46 82.7,54.46 U5.13 | U7.3 81.28,36.58 81.28,36.98 U7.4 81.28,37.19 80.67,37.8 v80.67,42.27 | 78.03,42.88 v78.44,42.47 | 78.03,42.88 77.22,42.88 U6.5 | 81.89,54.46 78.23,50.8 78.23,46.94 78.64,46.53 78.64,43.48 78.03,42.88
  Bottom 0.203: v80.67,42.27 80.47,42.47 v78.44,42.47
N$13
  Top 0.203: U5.14 82.91,54.86 84.94,54.86 84.94,51.82 87.17,49.58 87.99,49.58 U3.3
N$14  (via drill 0.25)
  Top 0.203: v84.94,44.3 82.91,44.3 U6.14
  Bottom 0.203: v84.94,44.3 90.02,49.38 90.02,50.8 Q1.C
N$15
  Top 0.203: U5.15 82.91,55.47 85.34,55.47 85.34,52.02 87.17,50.19 89.2,50.19 89.2,47.75 88.59,47.14 88.19,47.14 U3.5
N$16
  Top 0.203: U3.7 88.19,44.5 92.25,44.5 92.25,52.43 95.91,56.08 102.21,56.08 102.21,57.1 Q2.2
N$17  (via drill 0.25)
  Top 0.203: v81.48,44.91 82.7,44.91 U6.15
  Bottom 0.203: v81.48,44.91 96.11,59.54 102.21,59.54 Q2.3
N$18
  Top 0.203: R11.2 76.81,59.94 69.09,59.94 69.09,47.95 69.49,47.55 69.49,13.41 66.04,9.96 66.04,9.55 65.84,9.35 54.86,9.35 54.86,10.77 BRD1.JP2-54
N$19  (via drill 0.25)
  Top 0.203: R12.2 79.45,59.54 v79.45,58.12 | v68.68,47.35 68.28,46.94 68.28,12.8 65.63,10.16 65.63,9.75 56.49,9.75 56.49,10.77 BRD1.JP2-58
  Bottom 0.203: v68.68,47.35 v79.45,58.12
N$20
  Top 0.203: R9.2 109.93,33.12 112.17,33.12 112.17,32.51 112.37,32.31 114,32.31 114,34.95 100.79,48.16 100.79,48.56 99.97,49.38 97.13,49.38 97.13,40.84 96.52,40.23 95.1,40.23 U4.4
N$21  (via drill 0.25)
  Top 0.203: R7.2 103.02,33.73 v103.02,34.34 | v96.32,41.05 95.71,41.66 95.1,41.66 U4.2
  Bottom 0.203: v96.32,41.05 v103.02,34.34
N$22
  Top 0.203: R5.2 97.13,33.33 96.11,34.34 96.11,39.22 95.71,39.62 95.1,39.62 U4.5
N$23  (via drill 0.25)
  Top 0.203: v93.67,42.27 94.89,42.27 U4.1 | v91.64,40.23 87.78,36.37 87.78,34.75 R3.2
  Bottom 0.203: v91.64,40.23 v93.67,42.27
N$24
  Top 0.203: U4.12 100.58,39.62 99.57,39.62 99.57,35.56 101.19,33.93 101.19,32.51 100.99,32.31 94.49,32.31 94.49,31.09 93.67,30.28 91.44,30.28 91.44,33.33 92.66,34.54 R4.2
N$25
  Top 0.203: R6.2 100.18,33.33 99.16,34.34 99.16,40.23 99.77,40.84 100.58,40.84 U4.14
N$26  (via drill 0.25)
  Top 0.203: v106.48,34.34 106.48,33.53 106.68,33.33 R8.2 | v99.36,41.45 99.77,41.45 99.97,41.66 100.58,41.66 U4.15
  Bottom 0.203: v99.36,41.45 v106.48,34.34
N$27
  Top 0.203: R10.2 112.98,33.33 107.9,38.41 107.9,39.83 107.29,40.44 102.21,40.44 102.21,39.83 101.4,39.01 100.79,39.01 U4.11
N$28  (via drill 0.25)
  Top 0.203: 77.83,45.31 77.22,45.31 U6.1 77.83,45.31 | 77.83,45.31 78.03,45.31 78.23,45.11 78.23,44.3 77.22,44.3 U6.3 | v81.48,43.48 82.7,43.48 U6.13 | 77.83,45.31 v77.83,46.33
  Bottom 0.203: v81.48,43.48 78.64,46.33 v77.83,46.33
N$29
  Top 0.203: R13.2 83.11,60.15 82.3,60.96 82.3,68.68 83.52,69.9 83.52,72.34 83.11,72.75 76,72.75 76,67.87 67.87,59.74 67.87,18.49 65.63,16.26 65.63,16.05 61.57,11.99 57.3,11.99 57.3,10.97 BRD1.JP2-60
N$41  (via drill 0.25)
  Top 0.203: v77.83,38 78.64,37.19 U7.5 | v43.28,15.65 39.62,11.99 39.62,10.97 BRD1.JP2-16
  Bottom 0.203: v77.83,38 55.88,16.05 43.69,16.05 v43.28,15.65
N$42  (via drill 0.25)
  Top 0.203: v77.62,36.58 78.64,36.58 U7.6 | v42.06,13.41 40.44,11.79 40.44,10.97 BRD1.JP2-18
  Bottom 0.203: v77.62,36.58 56.69,15.65 44.3,15.65 v42.06,13.41
N$43  (via drill 0.25)
  Top 0.203: v77.83,33.73 77.83,35.76 78.64,35.76 U7.7 | v43.08,13.41 41.25,11.58 41.25,10.97 BRD1.JP2-20
  Bottom 0.203: v77.83,33.73 58.12,14.02 43.69,14.02 v43.08,13.41
N$141
  Top 0.203: U2.4 57.3,64.82 53.44,64.82 53.44,65.63 C8.1
N$143
  Top 0.203: C4.1 25.81,64.62 U1.4
N$144
  Top 0.203: R1.2 22.55,69.7 22.55,67.46 R2.1 22.55,67.26 22.55,63.6 C2.2 22.55,63.4 22.55,56.49 24.59,56.49 26.62,58.52 26.62,64.62 U1.5
N$185
  Top 0.381: BRD1.JP3-4 34.75,50.8 35.36,50.8 BRD1.JP3-6
RANGE_SEL_0
  Top 0.203: U4.10 100.79,38.41 102.01,38.41 102.01,31.09 79.45,8.53 53.24,8.53 53.24,10.77 BRD1.JP2-50
RANGE_SEL_1
  Top 0.203: U4.9 100.79,37.59 101.6,36.78 101.6,31.29 79.25,8.94 54.05,8.94 54.05,10.77 BRD1.JP2-52
RBIAS_N  (via drill 0.25)
  Top 0.203: U4.13 100.79,40.44 101.8,40.44 101.8,46.13 99.77,48.16 Q1.E | U3.2 90.83,50.8 v90.83,49.99
  Bottom 0.203: v90.83,49.99 92.46,48.36 99.57,48.36 Q1.E
RBIAS_P
  Top 0.203: U4.3 94.89,41.05 86.97,41.05 86.97,44.91 87.78,45.72 U3.6 88.39,45.72 91.64,48.97 91.64,52.43 95.5,56.29 95.5,57.1 99.57,57.1 Q2.1
REF_SEL
  Top 0.203: R13.1 83.31,61.98 87.58,66.24 87.58,71.12 S3.6

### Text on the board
tPlace: R | O | Y | G | BK | BR | SPI | PLATE | Opal Kelly XEM6010 | Intan Technologies | RHD2000 ELECTROPLATING | BOARD Version 1.0 | http://www.intantech.com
